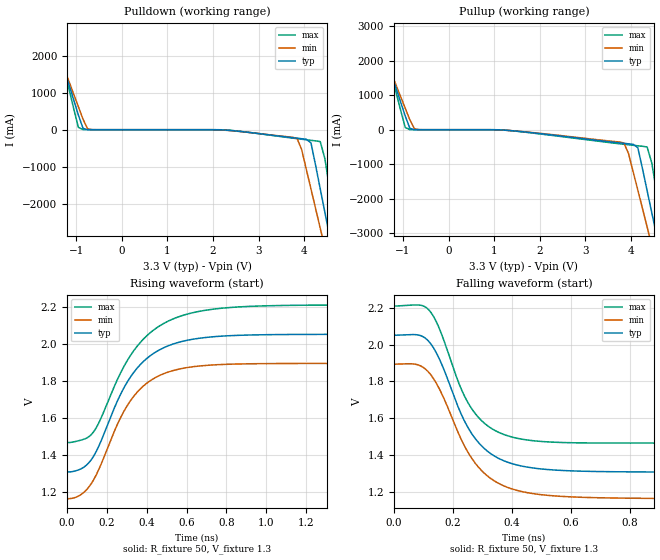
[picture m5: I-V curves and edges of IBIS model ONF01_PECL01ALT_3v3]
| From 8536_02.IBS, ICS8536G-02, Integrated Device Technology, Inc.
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[Model] ONF01_PECL01ALT_3v3
Model_type  Output_ECL
Polarity   Non-Inverting
Vmeas = 1.636
Rref = 50
Cref = 0
Vref = 1.3
|Variable  typ   min   max
C_comp   2p   1.5p   2.5p
[Voltage Range]   3.3   3.135   3.465
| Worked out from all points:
|   rising waveform, R_fixture 50, V_fixture 1.3: 20-80 % time 218ps typ, 206ps min, 242ps max; typ from 1.31 V to 2.05 V
|   falling waveform, R_fixture 50, V_fixture 1.3: 20-80 % time 134ps typ, 143ps min, 120ps max; typ from 2.05 V to 1.31 V
| Open source, no load
|  Voltage   I(typ)   I(min)   I(max)
[Pullup]
-3.3V     9.786A     8.45A      12.03A
-1.667V   3.247A     2.997A     3.691A
-1.565V   2.839A     2.657A     3.17A
-952.6mV  398mA      622.1mA    64.71mA
-850.5mV  36.63mA    284.2mA    1.532mA
-646.4mV  229.3uA    1.611mA    19.07uA
3.844V    -394.4mA   -383.6mA   -421.3mA
4.151V    -517.8mA   -1.749A    -465.4mA
4.355V    -1.764A    -2.812A    -500.3mA
4.559V    -3.036A    -3.875A    -1.773A
4.763V    -4.308A    -4.937A    -3.393A
6.6V      -15.79A    -14.52A    -18.03A
[Pulldown]
-3.3V     9.786A     8.45A      12.03A
-1.565V   2.839A     2.657A     3.17A
-1.463V   2.432A     2.317A     2.65A
-952.6mV  398mA      622.1mA    64.71mA
-850.5mV  36.63mA    284.2mA    1.532mA
-646.4mV  229.3uA    1.611mA    19.07uA
3.844V    -229.1mA   -232.1mA   -241.8mA
4.151V    -352.7mA   -1.598A    -286.7mA
4.355V    -1.599A    -2.66A     -322.1mA
4.559V    -2.871A    -3.722A    -1.595A
4.763V    -4.144A    -4.785A    -3.217A
6.6V      -15.69A    -14.41A    -17.97A
[Ramp]
|   typ   min   max
dV/dt_r   0.45V/0.37ns   0.45V/0.405ns   0.45V/0.27ns
dV/dt_f   0.45V/0.37ns   0.45V/0.405ns   0.45V/0.27ns
R_load =   50.0000
[Rising Waveform]
R_fixture = 50
V_fixture = 1.3   | VCC_typ - 2V
V_fixture_max = 1.465   | VCC_max - 2V
V_fixture_min = 1.135   | VCC_min - 2V
C_fixture = 0.0p
| Time   typ   min   max
0s        1.306V     1.161V     1.465V
70ps      1.323V     1.183V     1.479V
128ps     1.383V     1.254V     1.517V
258ps     1.703V     1.577V     1.819V
316ps     1.817V     1.689V     1.934V
398ps     1.919V     1.785V     2.042V
504ps     1.988V     1.846V     2.121V
658ps     2.03V      1.879V     2.175V
875ps     2.047V     1.891V     2.201V
2ns       2.052V     1.894V     2.211V
[Falling Waveform]
R_fixture = 50
V_fixture = 1.3   | VCC_typ - 2V
V_fixture_max = 1.465   | VCC_max - 2V
V_fixture_min = 1.135   | VCC_min - 2V
C_fixture = 0.0p
0s        2.052V     1.894V     2.211V
76ps      2.055V     1.893V     2.217V
118ps     2.018V     1.85V      2.19V
150ps     1.936V     1.772V     2.103V
222ps     1.644V     1.505V     1.782V
264ps     1.514V     1.38V      1.65V
326ps     1.409V     1.274V     1.549V
410ps     1.348V     1.21V      1.493V
708ps     1.309V     1.166V     1.465V
2ns       1.306V     1.161V     1.465V
